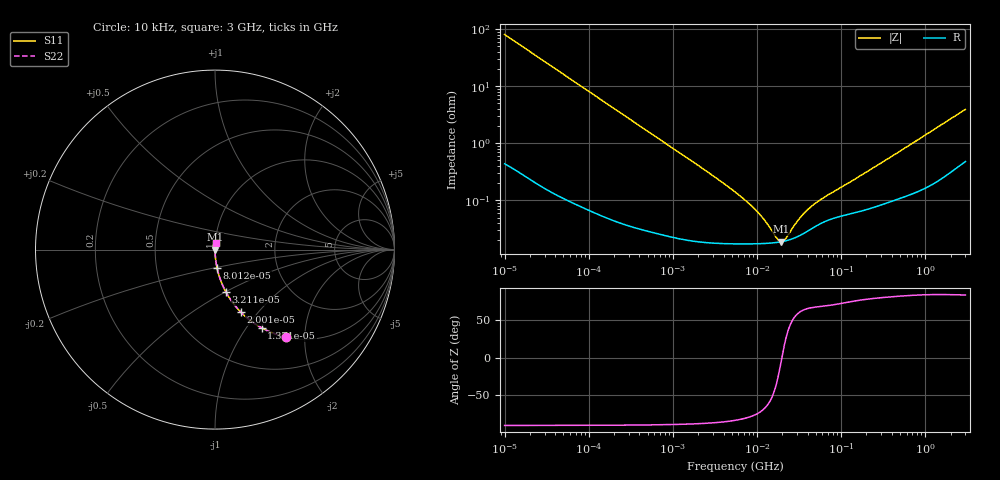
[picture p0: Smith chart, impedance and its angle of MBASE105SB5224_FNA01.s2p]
! MBASE105SB5224_FNA01  S-PARAMETER MODEL  ( Standard Model )
! Model Generated by TAIYO YUDEN Corporation (http://www.ty-top.com)
! Version 1.0
! TAIYO YUDEN Control No. 220601
! Copyright(c) 2013 TAIYO YUDEN CO.,LTD. All Rights Reserved.
! Product Description (link to TY-COMPAS)
! https://ds.yuden.co.jp/TYCOMPAS/or/detail?pn=MBASE105SB5224KFNA01&u=M
! Products Name : Multilayer Ceramic Capacitors
! Characteristics :
!  Capacitance : 0.22 [uF] , Rated Voltage : 16 [V] , TCC : X5R
!  Case Size : 1.0 x 0.5 / 0.039 x 0.02 [mm/inch] , Thickness : 0.5 / 0.02 [mm/inch]
!  (Conditions: Temperature = 25 [degC] , DC Bias Voltage = 0 [V])
! External Node Assignments :
!  1  o---| |---o  2
! GND o---------o GND
! Frequency Range : 10kHz  -  3GHz  [ 401 STEP ]
# MHZ S RI R 50
! Freq[MHz].  S11 Real  S11 Imag  S21 Real  S21 Imag  S12 Real  S12 Imag  S22 Real  S22 Imag
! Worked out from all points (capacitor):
!   401 points, 10 kHz to 3 GHz, reference 50 ohm
!   read as one part in series: C = 197 nF near 10.65 kHz
!   lowest |Z| = 18.9 mohm at 19.33 MHz (marker M1)
!   series resonance near 19.75 MHz, so ESL is about 330 pH
!   S11 on the Smith chart (normalised r, x): 10 kHz: 1.01, -1.62; 13.71 kHz: 1.01, -1.18; 20.01 kHz: 1.00, -0.81; 32.11 kHz: 1.00, -0.51; 80.12 kHz: 1.00, -0.20; 3 GHz: 1.01, +0.08
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0.01  0.396 -0.4864  0.604 0.4864  0.604 0.4864  0.396 -0.4864
0.013707  0.2599 -0.4358  0.7401 0.4358  0.7401 0.4358  0.2599 -0.4358
0.02001  0.1425 -0.3467  0.8575 0.3467  0.8575 0.3467  0.1425 -0.3467
0.03211  0.0614 -0.237  0.9386 0.237  0.9386 0.237  0.0614 -0.237
0.080117  0.011 -0.1005  0.989 0.1005  0.989 0.1005  0.011 -0.1005
0.082683  0.0104 -0.0974  0.9896 0.0974  0.9896 0.0974  0.0104 -0.0974
0.199902  0.0021 -0.0408  0.9979 0.0408  0.9979 0.0408  0.0021 -0.0408
0.683653  0.000401 -0.012  0.9996 0.012  0.9996 0.012  0.000401 -0.012
2.652321  0.00019 -0.00306  0.9998 0.00306  0.9998 0.00306  0.00019 -0.00306
5.477226  0.000175 -0.0014  0.9998 0.0014  0.9998 0.0014  0.000175 -0.0014
7.747855  0.000173 -0.000907  0.9998 0.000907  0.9998 0.000907  0.000173 -0.000907
9.97066  0.000174 -0.000621  0.9998 0.000621  0.9998 0.000621  0.000174 -0.000621
12.83117  0.000176 -0.000375  0.9998 0.000375  0.9998 0.000375  0.000176 -0.000375
17.04125  0.000183 -0.000125  0.9998 0.000125  0.9998 0.000125  0.000183 -0.000125
19.33182  0.000188 -1.81e-05  0.9998 1.81e-05  0.9998 1.81e-05  0.000188 -1.81e-05
20.5901  0.000191 3.52e-05  0.9998 -3.52e-05  0.9998 -3.52e-05  0.000191 3.52e-05
21.93027  0.000195 8.87e-05  0.9998 -8.87e-05  0.9998 -8.87e-05  0.000195 8.87e-05
32.0153  0.00024 0.000419  0.9998 -0.000419  0.9998 -0.000419  0.00024 0.000419
45.28751  0.000323 0.000737  0.9997 -0.000737  0.9997 -0.000737  0.000323 0.000737
64.06182  0.000426 0.00107  0.9996 -0.00107  0.9996 -0.00107  0.000426 0.00107
374.4521  0.00096 0.00548  0.999 -0.00548  0.999 -0.00548  0.00096 0.00548
3000  0.00626 0.0386  0.9937 -0.0386  0.9937 -0.0386  0.00626 0.0386
